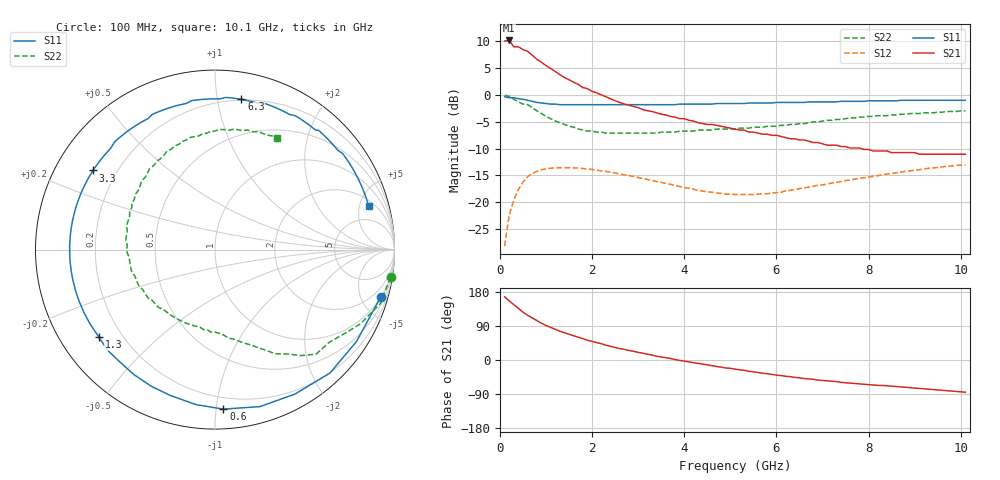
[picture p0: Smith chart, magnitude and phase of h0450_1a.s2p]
!HBFP-0450
!S and NOISE PARAMETERS at Vce=1V  Ic=1mA.  LAST UPDATED  09-04-98
# GHZ S MA R  50
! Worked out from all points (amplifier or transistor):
!   101 points, 100 MHz to 10.1 GHz, reference 50 ohm
!   highest |S21| = 10.1 dB at 200 MHz (marker M1)
!   |S21| within 3 dB of that: start of sweep to 732.8 MHz
!   unconditionally stable (mu >= 1): 3.239 GHz to end of sweep
!   at 1.7 GHz: K = 0.44, MSG = 7.8 dB, |S12| = -13.6 dB
!   at 5.1 GHz: K = 1.75, MAG = 1.1 dB, |S12| = -18.6 dB
!   at 10.1 GHz: K = 1.30, MAG = -2.3 dB, |S12| = -13.0 dB
!   lowest NFmin = 1.87 dB at 2 GHz
!   S11 on the Smith chart (normalised r, x): 100 MHz: 1.03, -6.97; 600 MHz: 0.12, -1.05; 1.3 GHz: 0.12, -0.33; 3.3 GHz: 0.11, +0.29; 6.3 GHz: 0.19, +1.17; 10.1 GHz: 2.56, +6.05
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0.1  0.96 -16.0  3.17 167.0  0.039 80.0  0.99 -9.0
0.2  0.94 -33.0  3.21 156.0  0.076 70.0  0.97 -18.0
0.3  0.94 -47.0  2.8 146.0  0.105 60.0  0.91 -27.0
0.4  0.92 -61.0  2.8 136.0  0.132 52.0  0.86 -33.0
0.5  0.91 -74.0  2.64 126.0  0.154 44.0  0.82 -39.0
0.6  0.89 -87.0  2.54 118.0  0.173 37.0  0.81 -46.0
0.8  0.85 -107.0  2.14 104.0  0.194 25.0  0.71 -55.0
0.9  0.84 -115.0  2.01 97.0  0.201 20.0  0.67 -60.0
1.1  0.82 -131.0  1.76 86.0  0.207 12.0  0.6 -66.0
1.3  0.81 -143.0  1.54 76.0  0.21 5.0  0.55 -72.0
1.8  0.81 -168.0  1.17 56.0  0.206 -9.0  0.47 -86.0
2.3  0.81 174.0  0.96 39.0  0.194 -20.0  0.44 -101.0
2.6  0.81 165.0  0.85 30.0  0.183 -24.0  0.44 -109.0
3.3  0.81 147.0  0.7 13.0  0.159 -33.0  0.44 -129.0
3.5  0.81 143.0  0.66 8.0  0.153 -34.0  0.45 -134.0
4.2  0.82 126.0  0.57 -7.0  0.132 -37.0  0.46 -151.0
5.1  0.83 106.0  0.48 -24.0  0.118 -34.0  0.48 -175.0
6.3  0.85 80.0  0.39 -44.0  0.129 -28.0  0.53 151.0
6.8  0.86 70.0  0.36 -51.0  0.141 -29.0  0.56 137.0
7.6  0.87 55.0  0.32 -61.0  0.161 -34.0  0.61 116.0
8.5  0.88 41.0  0.29 -69.0  0.185 -42.0  0.65 96.0
10.1  0.89 16.0  0.28 -85.0  0.223 -64.0  0.71 61.0
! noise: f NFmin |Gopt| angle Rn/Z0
1.8  1.95  0.68  154  0.1
2  1.87  0.72  164  0.06
2.5  2.27  0.75  -177  0.04
3.5  2.72  0.8  -147  0.29
4  3.01  0.83  -135  0.61
5  3.58  0.85  -110  1.77
5.5  3.93  0.87  -99  2.74
7  4.81  0.87  -67  6.48
8  4.83  0.89  -50  8.75
10  5.29  0.83  -18  9.99
